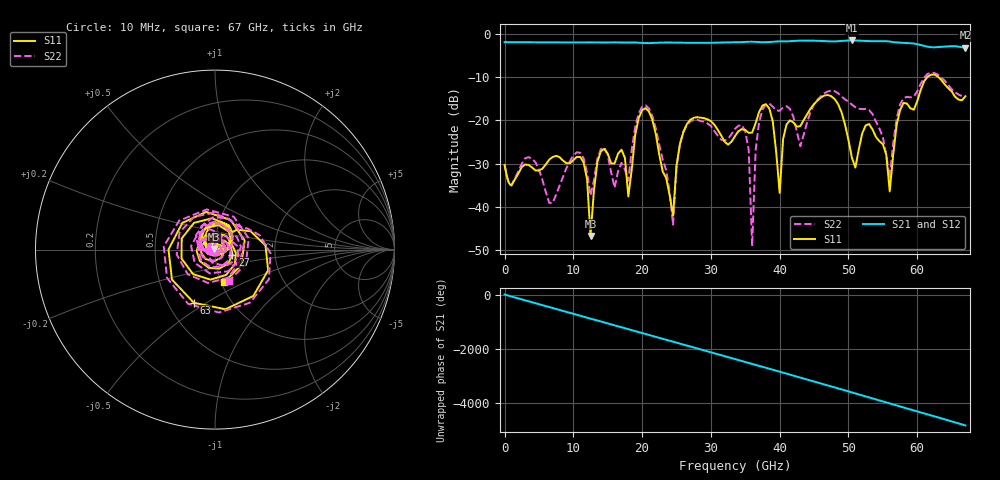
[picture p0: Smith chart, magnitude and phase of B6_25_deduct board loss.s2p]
!Keysight Technologies,N5247B,MY61255065,A.16.20.04
!Date: Monday, September 04, 2023 01:15:30
!Correction: S11(C  2-Port  )
!S21(C  2-Port  )
!S12(C  2-Port  )
!S22(C  2-Port  )
!S2P File: Measurements: S11, S21, S12, S22:
!Deduct Board Loss
# Hz S  dB  R 50
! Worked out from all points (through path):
!   142 points, 10 MHz to 67 GHz, reference 50 ohm
!   highest |S21| = -1.56 dB at 50.5 GHz (marker M1); lowest = -3.2 dB at 67 GHz (marker M2)
!   lowest |S11| = -46.7 dB at 12.5 GHz (marker M3), VSWR 1.01, Z = 49.6 + j0.295 ohm
!   |S11| at or under -10 dB: start of sweep to 61.48 GHz; 63.05 GHz to end of sweep
!   |S22| runs from -49.1 to -9.0 dB; largest |S21 - S12| = 0.0045
!   S11 on the Smith chart (normalised r, x): 10 MHz: 0.94, -0.00; 27 GHz: 1.21, -0.07; 63 GHz: 0.67, -0.44; 67 GHz: 1.03, -0.39
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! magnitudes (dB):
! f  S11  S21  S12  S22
! 10 MHz  -30.3  -2.0  -1.9  -30.4
! 11.5 GHz  -29.8  -2.0  -2.0  -28.8
! 12.5 GHz  -46.7  -2.0  -2.0  -37.4
! 14 GHz  -27.2  -2.0  -2.0  -26.7
! 20.5 GHz  -17.2  -2.2  -2.2  -16.6
! 22.5 GHz  -28.0  -2.1  -2.1  -25.7
! 24.5 GHz  -42.1  -2.0  -2.0  -44.1
! 27 GHz  -19.9  -2.1  -2.1  -20.3
! 34 GHz  -22.5  -2.0  -2.0  -21.3
! 35.5 GHz  -22.9  -1.9  -1.9  -26.9
! 36 GHz  -22.8  -1.9  -1.9  -49.1
! 36.5 GHz  -20.7  -1.9  -1.9  -27.0
! 37.5 GHz  -16.6  -2.0  -2.0  -17.5
! 40 GHz  -36.8  -1.8  -1.8  -17.8
! 41 GHz  -21.0  -1.8  -1.8  -16.7
! 45 GHz  -16.2  -1.6  -1.6  -16.3
! 50.5 GHz  -28.7  -1.6  -1.6  -16.4
! 53 GHz  -20.9  -1.7  -1.7  -17.7
! 56 GHz  -36.4  -1.8  -1.8  -33.3
! 57.5 GHz  -17.7  -2.1  -2.1  -16.4
! 63 GHz  -9.9  -3.1  -3.1  -9.4
! 67 GHz  -14.5  -3.2  -3.2  -14.4
